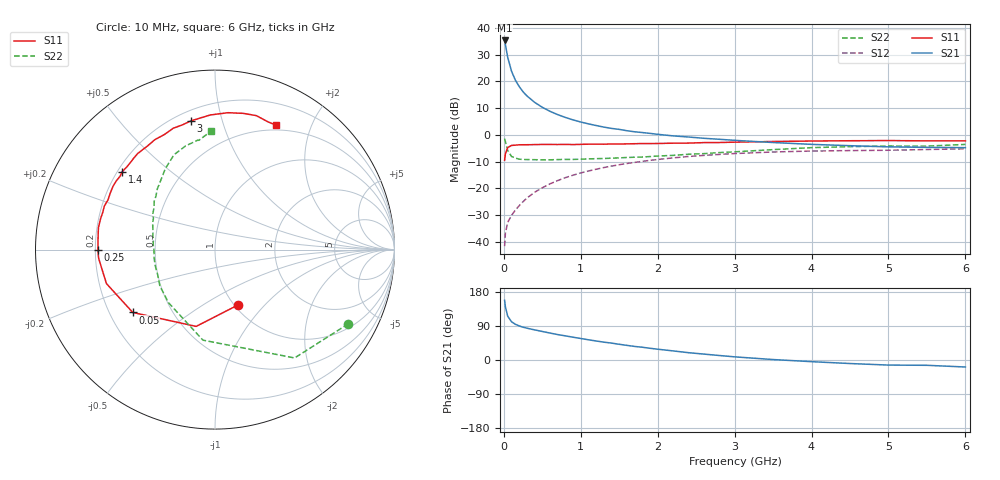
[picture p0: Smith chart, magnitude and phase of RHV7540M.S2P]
! SIEMENS Small Signal Semiconductors
! BFR106
! Si NPN RF Bipolar Junction Transistor in SOT23
! VCE = 0.75 V  IC = 40 mA
! Common Emitter S-Parameters:  August  1996
# GHz  S  MA  R  50
!  f  S11  S21  S12  S22
! GHz  MAG  ANG  MAG  ANG  MAG  ANG  MAG  ANG
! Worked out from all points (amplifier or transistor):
!   36 points, 10 MHz to 6 GHz, reference 50 ohm
!   highest |S21| = 35.4 dB at 10 MHz (marker M1)
!   |S21| within 3 dB of that: start of sweep to 29.4 MHz
!   unconditionally stable (mu >= 1): 215.5 MHz to end of sweep
!   at 250 MHz: K = 1.04, MAG = 19.4 dB, |S12| = -25.1 dB
!   at 1.4 GHz: K = 1.09, MAG = 5.3 dB, |S12| = -11.7 dB
!   at 6 GHz: K = 1.03, MAG = -0.8 dB, |S12| = -5.2 dB
!   S11 on the Smith chart (normalised r, x): 10 MHz: 1.04, -0.72; 50 MHz: 0.30, -0.31; 250 MHz: 0.21, -0.00; 1.4 GHz: 0.22, +0.35; 3 GHz: 0.26, +0.80; 6 GHz: 0.44, +1.52
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0.01  0.3341 -67.3  58.72 157.4  0.0082 74.0  0.8502 -29.1
0.02  0.4407 -103.8  49.47 140.7  0.0143 61.2  0.7491 -53.7
0.05  0.5767 -142.6  28.39 115.6  0.0229 50.0  0.509 -97.6
0.1  0.6337 -162.6  15.58 100.9  0.031 52.7  0.3932 -131.2
0.15  0.641 -171.4  10.56 94.2  0.0389 57.7  0.3678 -146.7
0.2  0.6504 -175.9  8.023 89.9  0.0471 61.3  0.3495 -155.6
0.25  0.6523 -179.7  6.407 86.5  0.0559 63.7  0.3456 -162.2
0.3  0.6524 177.8  5.367 84.0  0.0654 65.6  0.3443 -166.1
0.4  0.6563 172.8  4.072 79.5  0.0838 66.9  0.3422 -172.4
0.5  0.6609 169.3  3.281 75.3  0.1021 67.2  0.3402 -177.0
0.6  0.6604 165.1  2.76 71.1  0.1206 66.3  0.3404 179.9
0.7  0.659 161.5  2.392 67.1  0.1391 65.4  0.3439 177.1
0.9  0.6573 155.1  1.906 60.1  0.1756 62.6  0.3464 171.5
1.1  0.6688 148.1  1.606 53.3  0.2101 59.4  0.3548 167.5
1.4  0.6749 140.0  1.32 44.6  0.2596 54.0  0.3654 161.3
1.7  0.6822 131.3  1.141 35.8  0.3045 48.5  0.3809 155.1
2.2  0.6981 118.7  0.956 24.0  0.37 39.3  0.4123 145.5
3  0.7294 100.7  0.789 8.3  0.446 25.3  0.4804 130.1
3.5  0.7506 92.0  0.718 1.2  0.4775 17.6  0.5287 121.6
4.5  0.7752 78.3  0.626 -9.3  0.507 4.1  0.6005 105.8
5.5  0.7708 67.7  0.583 -14.0  0.5311 -4.0  0.6153 98.4
6  0.772 63.8  0.575 -18.5  0.5474 -10.2  0.6616 91.8
